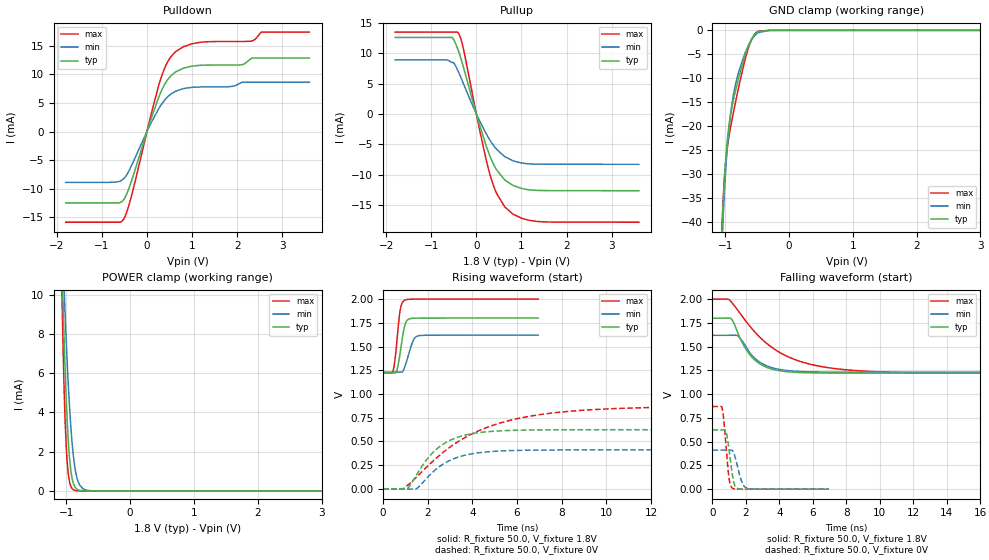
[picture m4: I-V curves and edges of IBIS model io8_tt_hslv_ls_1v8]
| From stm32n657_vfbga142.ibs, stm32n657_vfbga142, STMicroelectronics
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[Model]   io8_tt_hslv_ls_1v8
Model_type I/O
Polarity   Non-Inverting
Enable   Active-Low
| CAP_THRESHOLD on pad IOTT is "UDTCAPC" :
| Rising=30.0% of vddiov33m   Falling=70.0% of vddiov33m
| C_comp min and max val. don't necessarily correlate with the min and max pvt
| but are the smallest and greatest pad capacitance found.
| var   typ   min   max
C_comp   1.26678pF  1.09322pF  1.36432pF
|C_comp_pullup   869.30500fF  531.82500fF  521.20000fF
|C_comp_pulldown   397.47451fF  561.39043fF  843.11518fF
Vinl = 810.0mV
Vinh = 1.0V
Vmeas = 900.0mV   | Reference voltage for timing measurements
Cref  = 50.0pF   | Timing specification test load capacitance value
Rref  = 1.0MOhm   | Timing specification test load resistance value
Vref  = 990.0mV   | Timing specification test load voltage
[Model Spec]
| TIME_THRESHOLD on pin ZIV08M is "CMOS" :
| Rising=50.0% of vddv08m   Falling=50.0% of vddv08m
Vinl 675.70000mV 623.70000mV 735.70000mV
Vinh 1.12730V 1.01130V 1.24930V
| variable   typ   min   max
[Temperature Range] 25.0 125.0 -40.0
| variable   typ   min   max
[Voltage Range] 1.8V 1.62V 2.0V
| variable   typ   min   max
[POWER Clamp Reference] 1.8V 1.62V 2.0V
| variable   typ   min   max
[GND Clamp Reference] 0V 0V 0V
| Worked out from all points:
|   slope of the pulldown table from 0 to 0.27 V, typ, clamps not added: 43.9 ohm
|   slope of the pullup table from 0 to 0.27 V, typ, clamps not added: 42.7 ohm
|   GND clamp passes 1 mA (typ) near -0.55 V on its own axis
|   POWER clamp passes 1 mA (typ) near -0.93 V on its own axis
|   rising waveform, R_fixture 50.0, V_fixture 1.8V: 20-80 % time 235ps typ, 306ps min, 200ps max; typ from 1.22 V to 1.8 V
|   falling waveform, R_fixture 50.0, V_fixture 1.8V: 20-80 % time 1.26ns typ, 1.27ns min, 3.08ns max; typ from 1.8 V to 1.22 V
|   rising waveform, R_fixture 50.0, V_fixture 0V: 20-80 % time 1.45ns typ, 1.45ns min, 3.56ns max; typ from 0 V to 0.624 V
|   falling waveform, R_fixture 50.0, V_fixture 0V: 20-80 % time 294ps typ, 379ps min, 257ps max; typ from 0.624 V to 0 V
[POWER Clamp]
-1.8V     152.1mA    105.6mA    221.1mA
-1.07V    12.07mA    13.62mA    10.38mA
-1.05V    9.569mA    11.75mA    7.249mA
-1.03V    7.339mA    9.993mA    4.743mA
-1.01V    5.42mA     8.357mA    2.898mA
-990mV    3.841mA    6.859mA    1.662mA
-970mV    2.609mA    5.513mA    906.5uA
-940mV    1.358mA    3.806mA    344.1uA
-880mV    308.3uA    1.548mA    45.55uA
-790mV    28.47uA    298.6uA    2.144uA
-610mV    219.5nA    7.365uA    27.8nA
3.6V      0A         0A         0A
[GND Clamp]
-1.8V     -1.222A    -1.193A    -1.238A
-1.05V    -42.33mA   -45.55mA   -41.2mA
-1.04V    -38.89mA   -42.1mA    -37.88mA
-1.03V    -35.83mA   -38.98mA   -35.06mA
-1.01V    -30.7mA    -33.54mA   -30.61mA
-970mV    -23.47mA   -25.17mA   -24.97mA
-920mV    -18.06mA   -18.06mA   -20.63mA
-870mV    -14.51mA   -13.44mA   -17.13mA
-780mV    -9.532mA   -8.354mA   -11.38mA
-650mV    -3.743mA   -3.581mA   -4.327mA
-490mV    -324.1uA   -556uA     -259.6uA
3.6V      67.14nA    3.404uA    33.72nA
| variable   typ   min   max
[Pullup Reference] 1.8V 1.62V 2.0V
| variable   typ   min   max
[Pulldown Reference] 0V 0V 0V
[Pullup]
-1.8V     12.57mA    8.892mA    13.45mA
-670mV    12.57mA    8.892mA    13.45mA
-540mV    12.57mA    8.457mA    13.45mA
-390mV    10.19mA    6.793mA    13.18mA
-290mV    7.763mA    5.031mA    10.78mA
70mV      -1.782mA   -1.112mA   -2.559mA
320mV     -7.265mA   -4.527mA   -10.43mA
450mV     -9.207mA   -5.829mA   -13.09mA
630mV     -10.86mA   -7.029mA   -15.29mA
810mV     -11.75mA   -7.702mA   -16.46mA
1.37V     -12.57mA   -8.252mA   -17.68mA
3.6V      -12.62mA   -8.28mA    -17.79mA
[Pulldown]
-1.8V     -12.46mA   -8.882mA   -15.82mA
-520mV    -11.93mA   -8.267mA   -15.35mA
-350mV    -8.806mA   -6.088mA   -11.47mA
280mV     6.351mA    4.22mA     8.544mA
440mV     8.829mA    5.894mA    11.87mA
630mV     10.37mA    7.006mA    13.9mA
1.18V     11.56mA    7.771mA    15.57mA
1.8V      11.61mA    7.8mA      15.71mA
2.09V     11.64mA    8.54mA     15.71mA
2.32V     12.79mA    8.593mA    15.78mA
2.54V     12.82mA    8.593mA    17.35mA
3.6V      12.82mA    8.593mA    17.35mA
[Ramp]
dV/dt_r 374.38029mV/1.45079ns 246.6822mV/1.4465ns 522.26556mV/3.56384ns
dV/dt_f 347.15387mV/1.25875ns 233.36873mV/1.26724ns 468.14328mV/3.07825ns
R_load = 50.0
| Removed startup time: 0s 0s 0s  .
| Removed end time: 6.95ns.
[Rising Waveform]
R_fixture   = 50.0
V_fixture   = 1.8V
V_fixture_min = 1.62V
V_fixture_max = 2.0V
0s        1.221V     1.231V     1.22V
450ps     1.221V     1.231V     1.237V
500ps     1.222V     1.231V     1.296V
600ps     1.233V     1.231V     1.496V
750ps     1.403V     1.231V     1.853V
850ps     1.56V      1.23V      1.954V
1ns       1.741V     1.3V       1.991V
1.35ns    1.798V     1.561V     1.999V
1.6ns     1.799V     1.614V     1.999V
6.95ns    1.8V       1.62V      2V
| Removed startup time: 0s 0s 0s  .
| Removed end time: 199.9ns.
[Falling Waveform]
R_fixture   = 50.0
V_fixture   = 1.8V
V_fixture_min = 1.62V
V_fixture_max = 2.0V
0s        1.8V       1.62V      2V
1.1ns     1.8V       1.62V      1.977V
1.5ns     1.653V     1.618V     1.887V
2.2ns     1.423V     1.445V     1.724V
2.8ns     1.323V     1.341V     1.606V
3.5ns     1.267V     1.282V     1.499V
4.7ns     1.233V     1.245V     1.38V
6.3ns     1.223V     1.234V     1.298V
11.2ns    1.221V     1.231V     1.229V
199.9ns   1.221V     1.231V     1.22V
| Removed startup time: 0s 0s 0s  .
| Removed end time: 199.9ns.
[Rising Waveform]
R_fixture   = 50.0
V_fixture   = 0V
V_fixture_min = 0V
V_fixture_max = 0V
0s        252.6nV    3.541uV    371.3nV
900ps     -1.759mV   -890.1uV   1.91mV
1.1ns     3.503mV    -1.151mV   37.18mV
1.5ns     147.3mV    2.508mV    124.1mV
2.4ns     419.7mV    212.1mV    327mV
3.8ns     573.3mV    362.1mV    557.5mV
5.2ns     611.2mV    399.1mV    691mV
6.9ns     621.6mV    408.9mV    778.4mV
12ns      623.9mV    411.1mV    857.5mV
199.9ns   624mV      411.1mV    870.4mV
| Removed startup time: 0s 0s 0s  .
| Removed end time: 6.95ns.
[Falling Waveform]
R_fixture   = 50.0
V_fixture   = 0V
V_fixture_min = 0V
V_fixture_max = 0V
0s        624mV      411.1mV    870.4mV
550ps     624mV      411.1mV    870.7mV
600ps     623.9mV    411.1mV    838.6mV
800ps     612.7mV    411.1mV    486.7mV
1ns       408.3mV    411mV      107.8mV
1.2ns     145.2mV    407.3mV    9.993mV
1.4ns     16.95mV    308.1mV    1.826mV
1.75ns    1.2mV      80.52mV    678.3uV
2.05ns    631.3uV    10.46mV    424.6uV
6.95ns    21.23uV    40.7uV     36.77uV
